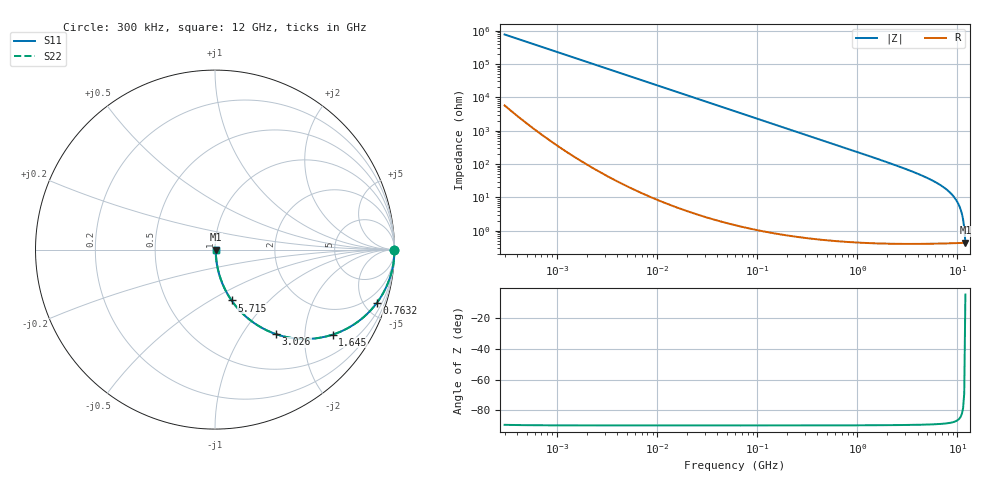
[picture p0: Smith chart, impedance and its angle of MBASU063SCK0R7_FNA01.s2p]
! MBASU063SCK0R7_FNA01  S-PARAMETER MODEL  ( Standard Model )
! Model Generated by TAIYO YUDEN Corporation (http://www.ty-top.com)
! Version 1.0
! TAIYO YUDEN Control No. 230609
! Copyright(c) 2023 TAIYO YUDEN CO.,LTD. All Rights Reserved.
! Product Description (link to TY-COMPAS)
! https://ds.yuden.co.jp/TYCOMPAS/or/detail?pn=MBASU063SCK0R7BFNA01&u=M
! Products Name : Multilayer Ceramic Capacitors
! Characteristics :
!  Capacitance : 0.7 [pF] , Rated Voltage : 50 [V] , TCC : CK / C0K
!  Case Size : 0.6 x 0.3 / 0.024 x 0.012 [mm/inch] , Thickness : 0.3 / 0.012 [mm/inch]
!  (Conditions: Temperature = 25 [degC] , DC Bias Voltage = 0 [V])
! External Node Assignments :
!  1  o---| |---o  2
! GND o---------o GND
! Frequency Range : 0.3MHz  -  12000MHz  [ 401 STEP ]
# MHZ S RI R 50
! Freq[MHz].  S11 Real  S11 Imag  S21 Real  S21 Imag  S12 Real  S12 Imag  S22 Real  S22 Imag
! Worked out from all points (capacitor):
!   401 points, 300 kHz to 12 GHz, reference 50 ohm
!   read as one part in series: C = 687 fF near 316.3 kHz
!   lowest |Z| = 437 mohm at 12 GHz (marker M1)
!   S11 on the Smith chart (normalised r, x): 300 kHz: open; 763.2 MHz: 1.01, -6.04; 1.645 GHz: 1.01, -2.76; 3.026 GHz: 1.01, -1.43; 5.715 GHz: 1.01, -0.63; 12 GHz: 1.01, -0.00
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0.3  1 -0.00013  9.78e-07 0.00013  9.78e-07 0.00013  1 -0.00013
1.769972  1 -0.000764  1.28e-06 0.000764  1.28e-06 0.000764  1 -0.000764
10.44266  1 -0.00451  2.2e-05 0.00451  2.2e-05 0.00451  1 -0.00451
60  0.9993 -0.0259  0.000681 0.0259  0.000681 0.0259  0.9993 -0.0259
164.1901  0.995 -0.0705  0.00504 0.0705  0.00504 0.0705  0.995 -0.0705
353.9943  0.977 -0.1494  0.023 0.1494  0.023 0.1494  0.977 -0.1494
763.2128  0.901 -0.298  0.099 0.298  0.099 0.298  0.901 -0.298
1135.593  0.8028 -0.3968  0.1972 0.3968  0.1972 0.3968  0.8028 -0.3968
1645.489  0.6556 -0.4737  0.3444 0.4737  0.3444 0.4737  0.6556 -0.4737
2088.533  0.5362 -0.4968  0.4638 0.4968  0.4638 0.4968  0.5362 -0.4968
3026.31  0.3403 -0.471  0.6597 0.471  0.6597 0.471  0.3403 -0.471
4270.516  0.1856 -0.3845  0.8144 0.3845  0.8144 0.3845  0.1856 -0.3845
5715.274  0.0927 -0.2836  0.9073 0.2836  0.9073 0.2836  0.0927 -0.2836
6879.757  0.0524 -0.2139  0.9476 0.2139  0.9476 0.2139  0.0524 -0.2139
7854.144  0.0317 -0.1632  0.9683 0.1632  0.9683 0.1632  0.0317 -0.1632
8732.115  0.0195 -0.1226  0.9805 0.1226  0.9805 0.1226  0.0195 -0.1226
9708.23  0.0111 -0.0821  0.9889 0.0821  0.9889 0.0821  0.0111 -0.0821
10236.47  0.00812 -0.0618  0.9919 0.0618  0.9919 0.0618  0.00812 -0.0618
10793.46  0.00603 -0.0416  0.994 0.0416  0.994 0.0416  0.00603 -0.0416
11083.22  0.0053 -0.0314  0.9947 0.0314  0.9947 0.0314  0.0053 -0.0314
11686.27  0.00445 -0.0113  0.9955 0.0113  0.9955 0.0113  0.00445 -0.0113
12000  0.00434 -0.000328  0.9957 0.000328  0.9957 0.000328  0.00434 -0.000328
